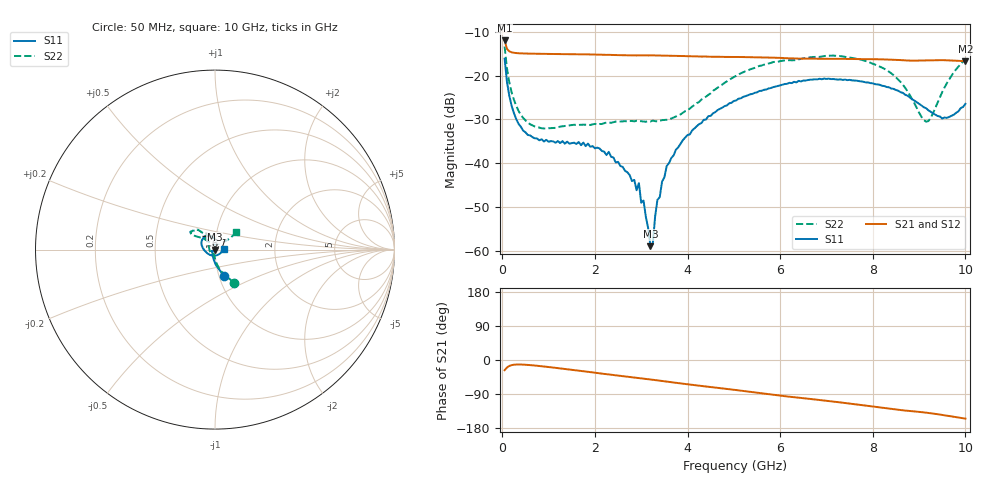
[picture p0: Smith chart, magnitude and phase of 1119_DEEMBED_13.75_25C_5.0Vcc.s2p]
!Hittite Microwave Corp.
!Digital Attenuator/PhaseShifter Rev 1.4.0
!Filename: C:\DATA\DATA\1119_DEEMBED_13.75_25C_5.0Vcc.s2p
!VNA ID: Agilent Technologies,N5224A,MY51441122,A.10.45.03
!Device type:
!2 Port Calibration.
!Temp(C): 25
!Lot Number:
!Serial Number:
!Operator:
!Misc:
!Attenuator:  13.750
# GHZ S DB R 50.0
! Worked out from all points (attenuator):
!   200 points, 50 MHz to 10 GHz, reference 50 ohm
!   highest |S21| = -11.96 dB at 50 MHz (marker M1); lowest = -16.7 dB at 10 GHz (marker M2)
!   lowest |S11| = -58.9 dB at 3.2 GHz (marker M3), VSWR 1.00, Z = 49.9 + j0.0359 ohm
!   |S11| at or under -10 dB: start of sweep to end of sweep
!   |S22| runs from -32.1 to -13.4 dB; largest |S21 - S12| = 0.00059
!   S11 on the Smith chart (normalised r, x): 50 MHz: 1.06, -0.32; 6.7 GHz: 0.90, +0.14; 10 GHz: 1.10, +0.01
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0.05  -16.12 -71.0  -11.96 -26.9  -11.96 -26.9  -13.35 -60.1
0.1  -21.35 -86.8  -13.88 -19.9  -13.87 -19.9  -18.25 -75.1
0.2  -26.82 -102.7  -14.66 -13.6  -14.66 -13.6  -23.75 -86.6
0.5  -32.92 -129.0  -14.94 -12.5  -14.95 -12.5  -30.20 -98.4
1.75  -35.28 -155.1  -15.13 -29.6  -15.13 -29.6  -31.18 -115.8
2.3  -37.39 -156.6  -15.24 -38.1  -15.24 -38.1  -30.71 -131.1
2.9  -46.16 -130.2  -15.38 -46.8  -15.39 -46.9  -30.31 -150.7
2.95  -44.53 -134.5  -15.36 -47.5  -15.37 -47.6  -30.38 -153.0
3  -49.02 -131.5  -15.36 -48.4  -15.37 -48.4  -30.39 -155.8
3.05  -48.52 -135.0  -15.37 -49.1  -15.38 -49.2  -30.47 -157.8
3.2  -58.93 161.4  -15.37 -51.4  -15.38 -51.4  -30.46 -165.3
3.25  -58.35 74.6  -15.37 -52.2  -15.38 -52.2  -30.25 -168.0
3.35  -48.35 58.6  -15.40 -53.8  -15.41 -53.8  -30.45 -173.3
3.4  -47.74 80.6  -15.39 -54.5  -15.40 -54.6  -30.30 -175.6
3.55  -40.63 70.8  -15.41 -57.1  -15.41 -57.1  -30.07 175.9
3.9  -34.71 65.6  -15.50 -62.5  -15.51 -62.6  -28.48 156.7
5.05  -25.67 83.9  -15.73 -79.3  -15.75 -79.4  -20.03 126.2
6.7  -20.90 123.6  -16.12 -103.4  -16.13 -103.4  -15.74 139.7
8.35  -22.66 166.9  -16.33 -128.1  -16.33 -128.2  -19.09 141.2
9.15  -27.42 -138.5  -16.51 -138.9  -16.52 -139.0  -30.50 91.3
9.5  -29.80 -83.2  -16.45 -145.0  -16.47 -145.0  -23.73 41.2
10  -26.44 4.6  -16.72 -154.7  -16.73 -154.7  -16.28 39.4
